(* Logix 5000 Rung export; software revision 16.04 *)

MODULES
   Local : vendor None type None code None
   MVI69E_AFC : vendor None type None code None
END_MODULES

TYPE AFCESiteAlarms :   // Indicates if a meter has any alarms
STRUCT
   Meter1 : BOOL;   // Meter in alarm
   Meter2 : BOOL;   // Meter in alarm
   Meter3 : BOOL;   // Meter in alarm
   Meter4 : BOOL;   // Meter in alarm
   Meter5 : BOOL;   // Meter in alarm
   Meter6 : BOOL;   // Meter in alarm
   Meter7 : BOOL;   // Meter in alarm
   Meter8 : BOOL;   // Meter in alarm
   Meter9 : BOOL;   // Meter in alarm
   Meter10 : BOOL;   // Meter in alarm
   Meter11 : BOOL;   // Meter in alarm
   Meter12 : BOOL;   // Meter in alarm
   Meter13 : BOOL;   // Meter in alarm
   Meter14 : BOOL;   // Meter in alarm
   Meter15 : BOOL;   // Meter in alarm
   Meter16 : BOOL;   // Meter in alarm
END_STRUCT
END_TYPE

TYPE AFCEMeterDifferentialGasBackPlaneReturn :   // Differential Gas Meter
STRUCT
   StandardDefault : AFCEMeterDifferentialGasStandardDataDflt;
   StandardRaw : INT[14];
   Extended : AFCEExtended;
END_STRUCT
END_TYPE

TYPE AFCEFlag :   // Flags contains status information updated by ladder and also trigger bits for clock update
STRUCT
   AFCStopped : BOOL;   // Indicates that the module has sent a new input block to be processed by ladder - UPDATED BY LADDER
   AFCInputSequenceNum : INT;   // Meter number (0 -15) associated to blocks 1-16. Used to update "Profile" (meter type and product group.) UPDATED BY LADDER
END_STRUCT
END_TYPE

TYPE AFCEUtilBlockNonInterrupt :
STRUCT
   Now : BOOL;
   ModbusMasterCommand : BOOL;
   ModbusMasterResponse : BOOL;
   Archive : DINT;
   Prover : BOOL;
   PassThru : BOOL;
   Calibration : BOOL;
END_STRUCT
END_TYPE

TYPE AFCEMeterDifferentialGasArchiveWrite :   // Write Archive
STRUCT
   Daily : BOOL;   // Set to 1 to write daily archive
   Hourly : BOOL;   // Set to 1 to write hourly archive
END_STRUCT
END_TYPE

TYPE AFCEMeterCalRequestActionType :
STRUCT
   ZeroShift : BOOL;   // Zero Shift
   SetZero : BOOL;   // Set Zero
   SetSpan : BOOL;   // Set Span
   SetMid1 : BOOL;   // Set Mid 1
   SetMid2 : BOOL;   // Set Mid 2
   SetMid3 : BOOL;   // Set Mid 3
END_STRUCT
END_TYPE

TYPE AFCEProveConfigEnable :   // Prove controls at enable
STRUCT
   MeterNumber : INT;   // Meter number requested (1-16)
   AutoAcceptProve : BOOL;   // Auto-accept the prove
   AutoContinueProve : BOOL;   // Auto-continue the prove
END_STRUCT
END_TYPE

TYPE AFCEModbusGateway :   // Modbus Gateway
STRUCT
   Command : AFCEModbusGatewayCommand[10];   // Modbus gateway commands - contains setup and modbus data
END_STRUCT
END_TYPE

TYPE AFCEMeterCalRequestActionValue :
STRUCT
   ZeroShift : AFCEMeterCalRequestValue;   // Zero Shift
   SetZero : AFCEMeterCalRequestValue;   // Set Zero
   SetSpan : AFCEMeterCalRequestValue;   // Set Span
   SetMid1 : AFCEMeterCalRequestValue;   // Set Mid 1
   SetMid2 : AFCEMeterCalRequestValue;   // Set Mid 2
   SetMid3 : AFCEMeterCalRequestValue;   // Set Mid 3
END_STRUCT
END_TYPE

TYPE AFCEMeterAnalysisError :
STRUCT
   StreamOutOfRange : BOOL;   // Requested Stream Number Out of Range
   StreamNotConfigured : BOOL;   // Requested Stream Not Configured
END_STRUCT
END_TYPE

TYPE AFCEMeterCalRequestValue :
STRUCT
   Applied : REAL;   // Applied
   Measured : REAL;   // Measured
END_STRUCT
END_TYPE

TYPE AFCEModbusMasterDataType :   // Modbus master data type
STRUCT
   Bit : BOOL;   // bit type
   Word : BOOL;   // word type (16-bit)
   Long : BOOL;   // long integer (32-bit)
   LongRemote : BOOL;   // long integer (32-bit)
END_STRUCT
END_TYPE

TYPE AFCEUtil :   // Used for internal ladder logic usage. These values must not be changed by user application.
STRUCT
   Flags : AFCEFlag;   // Wallclock update commands
   CycleCounter : INT;   // Reflects current block ID calculated by ladder to be sent to the module
   Buffer : AFCEUtilBuffer;
   Block : AFCEUtilBlock;
END_STRUCT
END_TYPE

TYPE AFCEWallclock :
STRUCT
   GetAFCTime : BOOL;   // Get current AFC Time
   SetAFCTimeFromPLCTime : BOOL;   // Set AFC time from PLC time. Updates current AFC time
   EnableLocalDateTime : BOOL;   // Enable Local Date Time.
   AFCTime : AFCETime;   // Coordinated Universal Time. Updated by either getting or setting AFC time.
END_STRUCT
END_TYPE

TYPE AFCEProvePhaseBitmap :   // AFC prove phase bitmap
STRUCT
   NotSelected : BOOL;   // Not selected
   Active : BOOL;   // Active, not counting
   CountingPast1stSwitch : BOOL;   // Counting past 1st switch for Udir and forward leg for Bdir)
   Past2ndSwitchFwdLeg : BOOL;   // Past 2nd switch forward leg (bidirectional only)
   Past1stSwithRetLeg : BOOL;   // Past 1st switch return leg (bidirectional only)
   RunComplete : BOOL;   // Run complete. past 2nd switch.
END_STRUCT
END_TYPE

TYPE AFCEProveInputConfig :   // Prove input block results - prover configuration
STRUCT
   Type : INT;   // Prover type
   Options : INT;   // Prover options
   RunsPerProveTotal : INT;   // Total runs per prove
   RunsPerProveSelected : INT;   // Selected runs per prove
   MaxRunsBeforeAbort : INT;   // Max total runs before abort
   ShortPassesPerRun : INT;   // Short passes per run if bidir = 2 , else 0
END_STRUCT
END_TYPE

TYPE AFCEMeterCalResponse :
STRUCT
   Trigger : BOOL;   // Send Error Code and Values to module to be recorded
   ErrorCode : SINT;   // Error Code to send. 0-4 allowed. 0=No error. 1-4=User defined.
   Value : AFCEMeterCalRequestValue;   // Value to Send
   Count : DINT;   // Number of calibration responses
END_STRUCT
END_TYPE

TYPE AFCEMeterDifferentialGasArchive :   // Different Gas Archive
STRUCT
   Write : AFCEMeterDifferentialGasArchiveWrite;
   Fetch : AFCEMeterDifferentialGasArchiveFetch;
END_STRUCT
END_TYPE

TYPE AFCEMeterDifferentialGasArchiveDflt :   // Default Configuration
STRUCT
   ClosingTimestamp : DINT;
   CumulativeActiveStreams : INT;
   CurrentActiveStream : SINT;
   MeterStatus : SINT;
   FlowingPeriod : DINT;
   PeriodDuration : DINT;
   AccumulatorTotalizer : DINT;
   AccumulatorResidue : REAL;
   MeterAlarms : DINT;
   PrimaryInput : REAL;   // Either Differential Pressure or Flow Rate
   Temperature : REAL;
   Pressure : REAL;
   RelativeDensity : REAL;
   ReferenceCompressibility : REAL;
   FlowingCompressibility : REAL;
   Fpv : REAL;
   PressureExtension : REAL;
   CoefficientDischarge : REAL;
   ExpansionFactor : REAL;
   Cprime : REAL;
   MassNRAccumulatorCurrent : REAL;   // Non-resettable
   MassNRAccumulatorOpening : REAL;   // Non-resettable
   EnergyNRAccumulatorCurrent : REAL;   // Non-resettable
   EnergyNRAccumulatorOpening : REAL;   // Non-resettable
   NetNRAccumulatorCurrent : REAL;   // Non-resettable
   NetNRAccumulatorOpening : REAL;   // Non-resettable
   GrossNRAccumulatorCurrent : REAL;   // Non-resettable
   GrossNRAccumulatorOpening : REAL;   // Non-resettable
   MolarFractionComponent01_C1 : REAL;
   MolarFractionComponent02_N2 : REAL;
   MolarFractionComponent03_CO2 : REAL;
   MolarFractionComponent04_C2 : REAL;
   MolarFractionComponent05_C3 : REAL;
   MolarFractionComponent06_H2O : REAL;
   MolarFractionComponent07_H2S : REAL;
   MolarFractionComponent08_H2 : REAL;
   MolarFractionComponent09_CO : REAL;
   MolarFractionComponent10_O2 : REAL;
   MolarFractionComponent11_IC4 : REAL;
   MolarFractionComponent12_NC4 : REAL;
   MolarFractionComponent13_IC5 : REAL;
   MolarFractionComponent14_NC5 : REAL;
   MolarFractionComponent15_C6 : REAL;
   MolarFractionComponent16_C7 : REAL;
   MolarFractionComponent17_C8 : REAL;
   MolarFractionComponent18_C9 : REAL;
   MolarFractionComponent19_C10 : REAL;
   MolarFractionComponent20_He : REAL;
   MolarFractionComponent21_Ar : REAL;
   UserDefinedFlowAverage1 : REAL;
   UserDefinedFlowAverage2 : REAL;
   UserDefinedFlowAverage3 : REAL;
END_STRUCT
END_TYPE

TYPE AFCEMeterDifferentialGasAlarm :   // Alarm Status and Control
STRUCT
   Control : AFCEMeterDifferentialGasAlarmControl;   // Alarm Control
END_STRUCT
END_TYPE

TYPE AFCEMeterDifferentialGasArchiveFetch :
STRUCT
   Daily : AFCEMeterDifferentialGasArchiveFetchT;
   Hourly : AFCEMeterDifferentialGasArchiveFetchT;
END_STRUCT
END_TYPE

TYPE AFCEMeterDifferentialGasAlarmControl :   // Differential Gas Process Alarm Control
STRUCT
   DifferentialPressure : AFCEMeterProcessAlarm;   // Differential Pressure Alarms
   FlowRate : AFCEMeterProcessAlarm;   // Flow Rate
   Temperature : AFCEMeterProcessAlarm;   // Temperature Alarms
   Pressure : AFCEMeterProcessAlarm;   // Pressure Alarms
END_STRUCT
END_TYPE

TYPE AFCEMeterArchiveFetchError :
STRUCT
   ArchiveSelectionInvalid : BOOL;   // Archive File Selection Invalid
   AgeOutsideSize : BOOL;   // Age Outside Configured File Size
   ArchiveNeverWritten : BOOL;   // Age OK but Archive Record Never Written (new or reconfigured meter)
   Reserverd1 : BOOL;
   Reserverd2 : BOOL;
   Reserverd3 : BOOL;
   Reserverd4 : BOOL;
   Reserverd5 : BOOL;
   Reserverd6 : BOOL;
   Reserverd7 : BOOL;
   Reserverd8 : BOOL;
   Reserverd9 : BOOL;
   Reserverd10 : BOOL;
   Reserverd11 : BOOL;
   Reserverd12 : BOOL;
   Reserverd13 : BOOL;
END_STRUCT
END_TYPE

TYPE AFCEModbusGatewayCommand :   // Modbus Gateway Command
STRUCT
   Config : AFCEModbusGatewayConfig;   // Config data to be entered by the user.
   Trigger : BOOL;   // Trigger the Command, when cleared module has responded.
   Data : INT[200];   // Contains modbus data written to the module (write commands)
END_STRUCT
END_TYPE

TYPE AFCEProveConfigAccept :   // Prove controls at accept. If auto-accept is selected must be available at enable
STRUCT
   RequestedInterpolationPoint : INT;   // Requested interpolation point (0 nearest)
   ApplyMFChangeAllStreams : BOOL;   // Apply change in meter factor to all streams
   ApplyMFChangeCurve : BOOL;   // Apply change in meter factor to all curve points
   ApplyNewMF : BOOL;   // CApply new meter factor
END_STRUCT
END_TYPE

TYPE AFCEModbusMasterCommand :   // Modbus Master Command
STRUCT
   Config : AFCEModbusMasterConfig;   // Modbus Master Configuration
   ErrorCode : INT;   // Error Code associated to Modbus Master Command
   Pending : BOOL;   // Pending Modbus Master Command - waiting for Modbus Response
   ReturnedTransactionID : DINT;   // Changes to Config.TransactionID value when response has returned.
   Data : INT[100];   // Read or Write Data
END_STRUCT
END_TYPE

TYPE AFCEMeterStatusMeter :   // Meter Status
STRUCT
   Enabled : BOOL;   // Meter Enable Status, 1=enabled
   EnableAlarm : BOOL;   // If set either: 1. The meter is not configured. 2. The event log is full, the action was not performed.
END_STRUCT
END_TYPE

TYPE AFCEMeterControl :   // Enable/Disable Meter and Streams
STRUCT
   Meter : AFCEMeterControlMeter;   // Control the Meter
   Stream : AFCEMeterControlStream;   // Control the Meter Streams
   ResetAccumulators : AFCEMeterSignals;   // Resets for meter accumulators
END_STRUCT
END_TYPE

TYPE AFCEProveSequencing :   // AFC prove sequencing tag for phase selection and ball positioning
STRUCT
   Phase : AFCEProvePhaseBitmap;   // AFC phase sequencing
   BallPositionReady : BOOL;   // Ball position: Ready (Udir & Bdir only; fwd leg Bdir)
   BallPositionSealed : BOOL;   // Ball position: Sealed (Udir & Bdir only; fwd leg Bdir)
   BallPositionReadyBwdLeg : BOOL;   // Ball position: Ready bwd leg (Bdir only)
   BallPositionSealedBwdLeg : BOOL;   // Ball position: Sealed bwd leg (Bdir only)
END_STRUCT
END_TYPE

TYPE AFCEMeterDifferentialGasArchiveFetchT :   // Fetch Archive
STRUCT
   Trigger : BOOL;   // Trigger Archive Fetch
   Age : INT;   // Initial Archive. 0 = Current Archive
   Error : AFCEMeterArchiveFetchError;   // Archive Fetch Error
   Default : AFCEMeterDifferentialGasArchiveDflt;   // Default Archive
   Raw : INT[100];   // Raw Archive
END_STRUCT
END_TYPE

TYPE AFCEUtilBlockInterrupt :
STRUCT
   Now : BOOL;
   ModbusGateway : DINT;
   EnableDisable : BOOL;
   Analysis : DINT;
END_STRUCT
END_TYPE

TYPE AFCEComponents :   // High precision gas component analysis (only supported version 2.07.000)
STRUCT
   C1 : REAL;   // Methane
   N2 : REAL;   // Nitrogen
   CO2 : REAL;   // Carbon Dioxide
   C2 : REAL;   // Ethane
   C3 : REAL;   // Propane
   H20 : REAL;   // Water
   H2S : REAL;   // Hydrogen Sulphide
   H2 : REAL;   // Hydrogen
   CO : REAL;   // Carbon Monoxide
   O2 : REAL;   // Oxygen
   IC4 : REAL;   // Iso-butane
   NC4 : REAL;   // Normal Butane
   IC5 : REAL;   // Iso-pentane
   NC5 : REAL;   // Normal-pentane
   C6 : REAL;   // Hexane
   C7 : REAL;   // Heptane
   C8 : REAL;   // Octane
   C9 : REAL;   // Nonane
   C10 : REAL;   // Decane
   He : REAL;   // Helium
   Ar : REAL;   // Argon
   NeoC5 : REAL;   // Not Used
   UxUser1 : REAL;   // Not Used
   UyUser2 : REAL;   // Not Used
   UxUser3 : REAL;   // Not Used
   UyUser4 : REAL;   // Not Used
   UxUser5 : REAL;   // Not Used
   UyUser6 : REAL;   // Not Used
   UxUser7 : REAL;   // Not Used
   UyUser8 : REAL;   // Not Used
   UxUser9 : REAL;   // Not Used
   UyUser10 : REAL;   // Not Used
END_STRUCT
END_TYPE

TYPE AFCEMeterStatus :   // Status
STRUCT
   Meter : AFCEMeterStatusMeter;   // Meter Status
   Stream : AFCEMeterStatusStream;   // Stream Status
END_STRUCT
END_TYPE

TYPE AFCEUtilBlock :
STRUCT
   ProcessInput : INT;
   InterruptPending : AFCEUtilBlockInterrupt;
   InterruptComplete : AFCEUtilBlockInterrupt;
   NonInterruptPending : AFCEUtilBlockNonInterrupt;
   NonInterruptComplete : AFCEUtilBlockNonInterrupt;
END_STRUCT
END_TYPE

TYPE AFCEModbusGatewayConfig :   // Modbus Ggateway Configuration
STRUCT
   Enable : BOOL;   // Set to 1 to enable modbus gateway command (0=disable)
   StartRegister : DINT;   // Start modbus address
   RegisterCount : INT;   // Word count (200 max)
   FunctionType : BOOL;   // 0 = read command, 1 = write command
   RegisterType : BOOL;   // 0 = holding register, 1 = input register
   SlaveType : BOOL;   // 0 = primary slave, 1 = virtual slave
END_STRUCT
END_TYPE

TYPE AFCEMeterControlMeter :   // Enable and Disable Meter
STRUCT
   Enable : BOOL;   // Enable the Meter
   Disable : BOOL;   // Disable the Meter
END_STRUCT
END_TYPE

TYPE AFCEMeterProfile :   // Meter configuration profile
STRUCT
   MeterType : BOOL;   // 0=Differential, 1=Linear
   ProductGroup : BOOL;   // 0=Gas, 1=Liquid
   PrimaryInput : BOOL;   // For differential, 0=Differential Pressure 1=Flow Rate. For Linear, 0=Pulse Count 1=Pulse Frequency
   AOIMismatch : BOOL;   // AOI Meter type does not match module for meter number
END_STRUCT
END_TYPE

TYPE AFCEModbusPassThru :   // AFC Modbus Pass-thru
STRUCT
   Enable : BOOL;   // Set to 1 to enable pass-thru functionality (requires AFC Manager setting)
   MessagePresent : BOOL;   // Message present in the response block
   GetMessage : BOOL;   // Get the pass-thru message. When the bit is cleared the message has been transferred to the PLC.
   FunctionBitWrite : BOOL;   // Function bit write
   OverflowError : BOOL;   // Overflow error flag
   ModbusAddress : INT;   // Destination modbus address
   RegisterCount : INT;   // Number of elements associated to command
   ReadDataWord : INT[125];   // Contains received data for word commands
   ReadDataBit : AFCEModbusPassThruBitData;   // Contains received data for bit commands
END_STRUCT
END_TYPE

TYPE AFCEUtilBuffer :   // Buffer
STRUCT
   Input : INT[248];   // Input buffer contains the complete block to be copied from the module
   Output : INT[247];   // Output buffer contains data the complete block to be copied to the module
   Process : INT[180];
   ArchiveDay : INT[98];
   ArchiveHour : INT[98];
   Prove : INT[26];
   Analysis : INT[198];
   MeterEnableDisable : INT[4];
   StreamEnable : INT[36];
   StreamDisable : INT[36];
   StreamSelect : INT[24];
   MeterSignals : INT[24];
   Calibration : INT[36];
END_STRUCT
END_TYPE

TYPE AFCEMeterDifferentialGasCalRequestProces :
STRUCT
   DifferentialPressure : BOOL;   // Differential Pressure
   Temperature : BOOL;   // Temperature
   Pressure : BOOL;   // Pressure
END_STRUCT
END_TYPE

TYPE AFCEProveStatus :   // Status of the prove (returned from the module to the processor)
STRUCT
   ProveAccepted : BOOL;   // Prove was accepted
   MeterFactorApplied : BOOL;   // Meter factor was applied
   MFAppliedToCurve : BOOL;   // Meter factor was applied to all points in the curve
   MFAppliedToStreams : BOOL;   // Meter factor was applied to all streams
   ProveRejectedByCommand : BOOL;   // Prove was rejected by command
   ProveRejectedNoRuns : BOOL;   // Prove was rejected - empty prove (no runs)
   ProveRejectedDivideBy0 : BOOL;   // Prove was rejected - divide by 0
   ProveEnabled : BOOL;   // Prove is enabled
   ProvingRunInProgress : BOOL;   // Proving run is in progress
   ProveRejectedAbort : BOOL;   // Prove rejected: abort
   ProvePaused : BOOL;   // Prove is paused
   RunCancelled : BOOL;   // Run Is cancelled
   RunTimedOut : BOOL;   // Run timed out
END_STRUCT
END_TYPE

TYPE AFCEMeterStatusStreamAlarm :   // Stream Alarms
STRUCT
   StreamOutOfRange : BOOL;   // Requested Stream Number Out of Range
   StreamNotConfigured : BOOL;   // Requested Stream not Configured
   StreamNotEnabled : BOOL;   // Requested Stream not Enabled
   EventLogFull : BOOL;   // Event Log Full, Action not Performed
END_STRUCT
END_TYPE

TYPE AFCEMeterDifferentialGasCalRequest :
STRUCT
   ProcessVariable : AFCEMeterDifferentialGasCalRequestProces;   // Process Variable
   ActionType : AFCEMeterCalRequestActionType;   // Action Type
   Value : AFCEMeterCalRequestActionValue;   // Value
   Count : DINT;   // Number of calibration requests
END_STRUCT
END_TYPE

TYPE AFCEProveConfig :   // Controls (configuration settings) associated to the prover
STRUCT
   Enable : AFCEProveConfigEnable;   // Controls at enable
   Accept : AFCEProveConfigAccept;   // Controls at accept
END_STRUCT
END_TYPE

TYPE AFCESiteStatus :   // Site status bits - contains general information about the module - not meter specific
STRUCT
   AFCActive : BOOL;   // AFC active
   ChecksumAlarms : BOOL;   // Checkum alarm active
   Reserved2 : BOOL;
   Reserved3 : BOOL;
   PLCHalted : BOOL;   // PLC in program mode or missing
   CfgChanged : BOOL;   // Configuration changed
   Powerup : BOOL;   // Module powered up
   ColdStart : BOOL;   // Module performed cold start (BBRAM initialized)
   ModbusMasterPending : BOOL;   // Modbus Master Poll Pending
   ModbusMasterComplete : BOOL;   // Modbus Master Poll Complete
   ModbusPassThruPending : BOOL;   // Modbus Pass-thru Input Pending
   CalibrationRequest : BOOL;   // Calibration request from module
   ProverEnabled : BOOL;   // Prover Enabled
   Reserved13 : BOOL;
   Reserved14 : BOOL;
   Reserved15 : BOOL;
END_STRUCT
END_TYPE

TYPE AFCEMeterDifferentialGasStandardDataDflt :   // EAFC Backplane Return Standard Data
STRUCT
   Meter_Alarms : DINT;   // Meter alarms
   NR_Acc_Net_Totalizer : DINT;   // Non-resettable accumulator, net, totalizer (m3)
   NR_Acc_Net_Residue : REAL;   // Non-resettable accumulator, net, residue (m3)
   FlowRate_Net : REAL;   // Flow rate, net (m3/h)
   FlowRate_Gross : REAL;   // Flow rate, gross (m3/h)
   Ifpv : REAL;   // AGA 8, Supercompressibility, Fpv
   Cprime : REAL;   // C-prime
END_STRUCT
END_TYPE

TYPE AFCEModbusMaster :   // Modbus Master. Port 3 must be configured as modbus master through AFC Manager to use this feature.
STRUCT
   Enable : BOOL;   // Enable the modbus master funcionality
   CommandIndex : INT;   // Selects which command index will be executed
   Command : AFCEModbusMasterCommand[10];   // Each command contains a specific modbus request to be sent out of the port
END_STRUCT
END_TYPE

TYPE AFCEProveProcess :   // Prove process output from processor to the module
STRUCT
   Sequencing : AFCEProveSequencing;   // Prover sequencing
   Temperature : REAL;   // Temperature for Single Probe provers. And Inlet Temperature for Dual Probe Provers.
   OutletTemperature : REAL;   // Outlet Temperature for Provers with Dual Probes.
   SwitchBarTemperature : REAL;   // Switch bar temperature
   Pressure : REAL;   // Pressure for Single Probe provers. And Inlet Pressure for Dual Probe Provers.
   OutletPressure : REAL;   // Outlet Pressure for Provers with Dual Probes.
   ProverDensity : REAL;   // Prover density
END_STRUCT
END_TYPE

TYPE AFCEExtended :
STRUCT
   Trigger : BOOL;
   Data : AFCEExtendedData;
END_STRUCT
END_TYPE

TYPE AFCEMeterSignals :   // Meter trigger accumulator and archive resets
STRUCT
   ResetAccumulator1 : BOOL;   // Set to 1 to reset resettable accumulator 1
   ResetAccumulator2 : BOOL;   // Set to 1 to reset resettable accumulator 2
   ResetAccumulator3 : BOOL;   // Set to 1 to reset resettable accumulator 3
   ResetAccumulator4 : BOOL;   // Set to 1 to reset resettable accumulator 4
END_STRUCT
END_TYPE

TYPE AFCEMeterProcessAlarm :   // Process Alarms
STRUCT
   SetGeneralFail : BOOL;   // Set to indicate General Failure of the Transmitter
   StaleData : BOOL;   // Clear to Indicate new process input data
   SetLowThreshold : BOOL;   // Set to indicate Lower Range Limit Exceeded
   SetHighThreshold : BOOL;   // Set to indicate Upper Range Limit Exceeded
   SetAutoClearStaleData : BOOL;   // Set to automatically clear stale data
END_STRUCT
END_TYPE

TYPE AFCETime :   // AFC time format used for wallclock update.
STRUCT
   Year : DINT;   // Year
   Month : DINT;   // Month
   Day : DINT;   // Day
   Hour : DINT;   // Hour
   Minute : DINT;   // Minute
   second : DINT;   // Seconds
END_STRUCT
END_TYPE

TYPE AFCEModbusMasterSwap :   // Modbus master swap words/ swap bytes
STRUCT
   SwapWords : BOOL;   // Swap words
   SwapBytes : BOOL;   // Swap bytes
END_STRUCT
END_TYPE

TYPE AFCEMeterControlStream :
STRUCT
   Selected : SINT;   // Stream to Enable or Disable and/or make active.
   EnableSelected : BOOL;   // Enable the Selected Stream
   DisableSelected : BOOL;   // Disable the Selected Stream
   SetSelectedToActive : BOOL;   // Set Selected to Active Stream
END_STRUCT
END_TYPE

TYPE AFCEProvePulseCount :   // Values to be supplied at the end of the pass/run
STRUCT
   Meter : DINT;   // Meter pulse count
   MasterMeter : DINT;   // Master meter pulse count
END_STRUCT
END_TYPE

TYPE AFCEMeterDifferentialGasCal :   // Processor Mediated Calibration
STRUCT
   Request : AFCEMeterDifferentialGasCalRequest;   // Calibration Request from module
   Response : AFCEMeterCalResponse;   // Processor Response
END_STRUCT
END_TYPE

TYPE AFCEMeterStatusStream :
STRUCT
   Active : INT;   // Current Active Stream
   Enabled : AFCEMeterStatusStreamEnabled;   // Enabled Streams
   Configured : AFCEMeterStatusStreamEnabled;   // Configured Streams
   EnableAlarm : AFCEMeterStatusStreamAlarm;   // Enable Alarms
END_STRUCT
END_TYPE

TYPE AFCEExtendedData :
STRUCT
   Raw : INT[64];
END_STRUCT
END_TYPE

TYPE AFCEMeterDifferentialGasProcess :   // Differential Gas Process Variables
STRUCT
   DifferentialPressure : REAL;   // Differential pressure if Primary Input = Differential pressure
   FlowRate : REAL;   // Flow Rate if Primary Input = Flow Rate
   Temperature : REAL;   // Temperature
   Pressure : REAL;   // Static pressure
END_STRUCT
END_TYPE

TYPE AFCEModbusPassThruBitData :   // AFC Modbus Pass-thru Bit Data
STRUCT
   Data : BOOL[2016];   // Contains received data for bit commands
END_STRUCT
END_TYPE

TYPE AFCEModbusMasterConfig :   // Modbus master command settings
STRUCT
   Enable : BOOL;   // Set to 1 to enable command (0=disable)
   FunctionType : BOOL;   // Set to 1 to select write command (0=read command)
   RegisterBank : BOOL;   // Set to 1 to select input register (0=holding register)
   DataType : AFCEModbusMasterDataType;   // Select data type format
   SwapOption : AFCEModbusMasterSwap;   // Select byte and word swap (1 = swap, 0 = no swap)
   TypeSwap : INT;   // This value is calculated by ladder logic and must not be modified by user
   SlaveAddress : INT;   // Modbus slave address of remote device
   ModbusAddress : INT;   // Modbus data address on remote slave
   ElementCount : INT;   // Number of data elements (125 words)
   TransactionID : INT;   // Transaction ID. This value is returned to the ReturnedTransaction ID when the response has been received.
END_STRUCT
END_TYPE

TYPE AFCEModuleDef :   // Main user defined data type
STRUCT
   ModbusGateway : AFCEModbusGateway;   // Reads and write data between processor and module modbus table
   ModbusMaster : AFCEModbusMaster;   // Setup modbus master commands to be sent to remote slaves (through Port 3)
   ModbusPassThru : AFCEModbusPassThru;   // Modbus pass-thru data
   SiteStatus : AFCESiteStatus;   // Site status
   MeterAlarms : AFCESiteAlarms;   // Meter Alarms
   Prove : AFCEProve;   // Prover
   Wallclock : AFCEWallclock;   // Set clock and get clock information
   Firmware : AFCEFirmwareVersion;   // Firmware information
   Util : AFCEUtil;   // Used by ladder logic
END_STRUCT
END_TYPE

TYPE AFCEMeterDifferentialGas :   // Differential Gas Meter
STRUCT
   Control : AFCEMeterControl;   // Meter Control
   Status : AFCEMeterStatus;   // Meter Status
   ProcessVariables : AFCEMeterDifferentialGasProcess;   // Input process variables to be transferred to the module
   Analysis : AFCEMeterAnalysis;   // Molar Analysis data to be transferred to the module (only for gas products with online gas chromatograph applications)
   Alarm : AFCEMeterDifferentialGasAlarm;   // Meter Alarm status and control
   Archive : AFCEMeterDifferentialGasArchive;   // Archive
   Profile : AFCEMeterProfile;   // Module profile (meter type/product group) transfered from the module
   Calibration : AFCEMeterDifferentialGasCal;   // Calibration
   BackPlaneReturn : AFCEMeterDifferentialGasBackPlaneReturn;
END_STRUCT
END_TYPE

TYPE AFCEMeterAnalysis :   // Meter analysis components. Allows the processor to update molar analysis for low precision and high precision streams.
STRUCT
   Trigger : BOOL;   // Set to 1 to Send Updated Component Data to the Module
   Stream : INT;   // Stream for Analysis. Select 0 for current active stream.
   Error : AFCEMeterAnalysisError;   // Analysis Error
   Components : AFCEComponents;   // High precision gas components (floating point per component). Only supported for firmware version 2.07.000 or later
END_STRUCT
END_TYPE

TYPE AFCEProveSignals :   // Contains the proving signals that will trigger specific tasks from the module
STRUCT
   EnableProve : BOOL;   // Enables the prove
   AcceptProve : BOOL;   // Accepts the prove
   RejectProve : BOOL;   // Reject the prove
   RunStart : BOOL;   // Starts the run
   RunComplete : BOOL;   // Flags that the run is complete
   RunCancel : BOOL;   // Cancels the run
   RunDelete : BOOL;   // Deletes the run
   PassComplete : BOOL;   // Flag that the pass is complete
   PauseProve : BOOL;   // Pauses the Proving Process
   AbortProve : BOOL;   // Aborts the prove
END_STRUCT
END_TYPE

TYPE AFCEFirmwareVersion :
STRUCT
   Major : SINT;   // Major Version number
   Minor : SINT;   // Minor Version number
   Revision : INT;   // Revision
END_STRUCT
END_TYPE

TYPE AFCEProveRunResults :   // Run results of the prove. Copied from the module to the pocessor
STRUCT
   CountAttempted : INT;   // Run count attempted
   CountCompleted : INT;   // Run count completed
   CountSelected : INT;   // Run count selected
   RunsSelected : INT;   // Bit Mapped Runs selected for calculations from completed runs
   NewMeterFactor : REAL;   // New meter factor
   ChangeInMeterFactor : REAL;   // Change in meter factor
END_STRUCT
END_TYPE

TYPE AFCEMeterStatusStreamEnabled :   // Stream Status 1 = Enabled
STRUCT
   Stream1 : BOOL;
   Stream2 : BOOL;
   Stream3 : BOOL;
   Stream4 : BOOL;
   Stream5 : BOOL;
   Stream6 : BOOL;
   Stream7 : BOOL;
   Stream8 : BOOL;
   Stream9 : BOOL;
   Stream10 : BOOL;
   Stream11 : BOOL;
   Stream12 : BOOL;
   Stream13 : BOOL;
   Stream14 : BOOL;
   Stream15 : BOOL;
   Stream16 : BOOL;
END_STRUCT
END_TYPE

TYPE AFCEProve :   // Prove
STRUCT
   Process : AFCEProveProcess;   // Process Variables
   Signals : AFCEProveSignals;   // AFC Prove Signals (triggers the proving update)
   Config : AFCEProveConfig;   // AFC Prove Control (configuration settings)
   PulseCounts : AFCEProvePulseCount;   // Pulse counts to be updated at the end of the run/pass
   ConfigInput : AFCEProveInputConfig;   // AFC prover input configuration
   Status : AFCEProveStatus;   // AFC prover status
   ErrorCode : INT;   // Prove error code
   ProveControlsEcho : INT;   // AFC module Echos the state of the Prove Controls
   RequestedMeterEcho : INT;   // AFC module Echos the Meter number requested
   RequestedCurvePointEcho : INT;   // AFC module Echos the requested Curve Point
   RunResults : AFCEProveRunResults;   // Prove and run results
   ProveEnabled : BOOL;   // ON if prove is enabled. This flag is coped from inputbuffer[247]
END_STRUCT
END_TYPE

ADD_ON_INSTRUCTION AOI69EAFCMeterDifferentialGas   (* revision 1.6, vendor ProSoft Technology Inc., ExecutePrescan *)
// Add-On instruction for the MVI69E-AFC.
// Differential Gas Meter
// Revision note:
// Updated  BackplaneReturn Tag name from ProcessInputs to Standard
// and ComponentAnalysis to Extended
// Help:
// AOI69EAFCMeterDifferentialGas v1.1
// Compatible with version 4.04 of MVI69E-AFC firmware or higher.
// v1.1 Comp Analysis Return fix
// v1.2 Added Flow Rate Process Input and Flow Rate Alarm Controller Tags for Flow Rate Devices (and not just for Differential Pressure)
// v1.3: Addition of default process input backplane return data mapping..
// v1.4: Changed Prescan FLL instruction length from 240 words to 180 for proccess inputs. This stopped mismatch issue
// v1.4:  Made correlation changes between the Module Archive Default UDTs and the AOI Archive Default UDTs.
// v1.5: Made changes to the Flow Rate Primary Input Block ID Insertion in Rung 8 (Removed +1), Modified ProcessInputBlockID Tag Data Type from DINT to INT and modified ModbusGatewayConfig UDT StartRegister Tag Data Type from INT to DINT.
// v1.6: Updated Tags names AFCMeterXXYYYYYY.BackPlaneReturn.ProcessInputs to
// AFCMeterXXYYYYYY.BackPlaneReturn.Standard and
// AFCMeterXXYYYYYY.BackPlaneReturn.ComponentAnalysis
//  to AFCMeterXXYYYYYY.BackPlaneReturn.Extended.
VAR_IN_OUT
   ConnectionInput : INT[248]; {required}
   AFC : AFCEModuleDef; {required}
   AFCMeter : AFCEMeterDifferentialGas; {required}
END_VAR
VAR_INPUT
   MeterNumber : SINT; {required}   // Meter Number Set to a number between 1 and 16
END_VAR
VAR
   TimestampBuffer : DINT;
   StreamSelectedShift : DINT;
   StreamSelectBuffer : INT;
   EnabledStatusBuffer : INT;
   StreamSelectBlockID : DINT;
   StreamNumberShift : DINT;
   StreamErrorBuffer : DINT;
   StreamEnableBlockID : DINT;
   StreamEnableBitPosition : DINT;
   StreamDisableBlockID : DINT;
   ProfileBuffer : SINT[2];
   ProcessInputBlockID : DINT;
   CalibrationHandleBuffer : INT;
   AnalysisGroupBitPosition : INT;
   ProcessAlarmShifter : DINT;
   ProcessAlarmBuffer : DINT;
   MeterSignaltBlockID : DINT;
   MeterNumberShift : DINT;
   MeterNumberBitPostition : DINT;
   Inputbuffer : INT[248];
   CurrentHourlyAgeONS : BOOL;
   CurrentHourlyAge : DINT;
   CurrentDailyAgeONS : BOOL;
   CurrentDailyAge : DINT;
   ClearMeterSignal : BOOL;   // Repeat the meter signal block with cleared signal bits. This allows repeat triggering of a signal.
   CalibrationMeterNumberBuffer : DINT;
   CalibrationMediationPending : BOOL;
   CalibrationInputScalingIndex : DINT;
   AnalysisErrorBuffer : INT;
   ArchiveStream : DINT;
   ArchiveMeterStatusRaw : DINT;
   ArchiveMeterStatusActiveStream : DINT;
   ArchiveHourlyRawSize : DINT;
   ArchiveHourlyOffset : DINT;
   ArchiveHourlyDefaultSize : DINT;
   ArchiveDailyRawSize : DINT;
   ArchiveDailyOffset : DINT;
   ArchiveDailyDefaultSize : DINT;
   ArchiveCompleteBitCheck : DINT;
   ArchiveBlockID : DINT;
   AnalysisGroupShift : DINT;
   AnalysisCompleteBitCheck : DINT;
   AnalysisBufferOffset : DINT;
   AnalysisBlockID : DINT;
   AFCStopped : BOOL;
   AFCInputDataAvailable : BOOL;
END_VAR

ROUTINE Logic   (* ladder *)
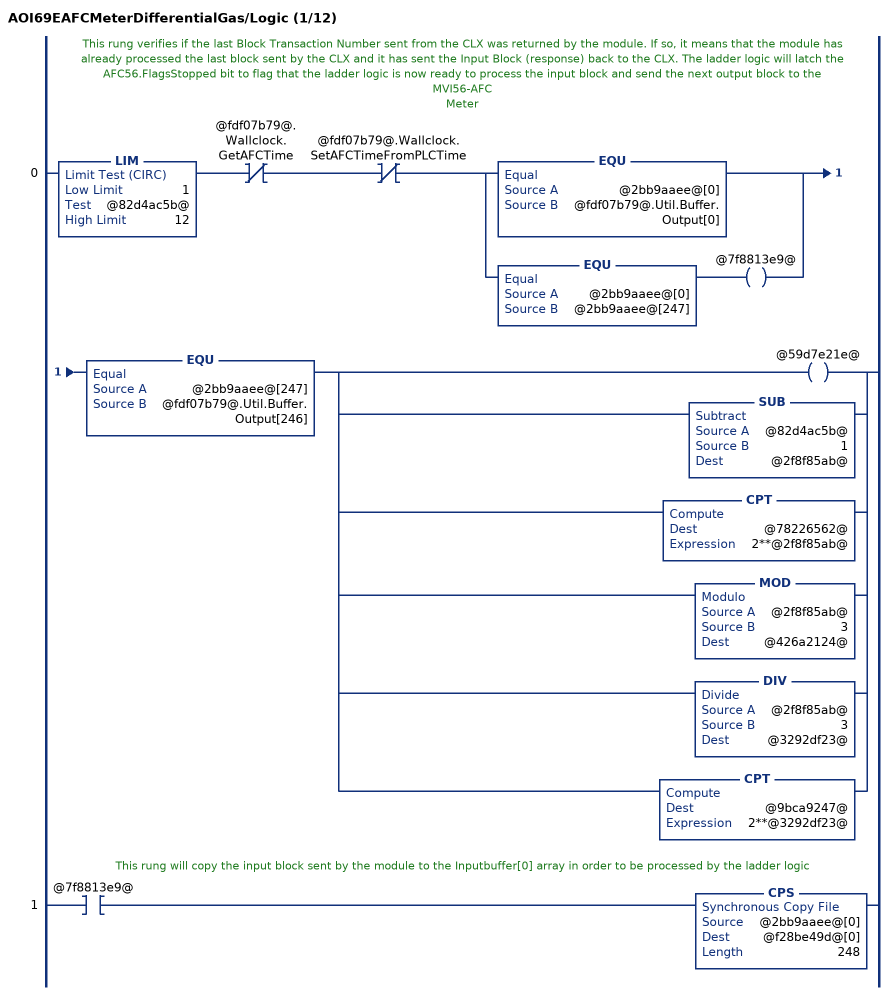
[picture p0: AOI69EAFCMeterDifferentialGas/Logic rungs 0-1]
   // This rung verifies if the last Block Transaction Number sent from the CLX was returned by the module. If so, it means that the module has already processed the last block sent by the CLX and it has sent the Input Block (response) back to the CLX. The ladder logic will latch the AFC56.FlagsStopped bit to flag that the ladder logic is now ready to process the input block and send the next output block to the MVI56-AFC
   // Meter
   0: LIM(1,@82d4ac5b@,12)XIO(@fdf07b79@.Wallclock.GetAFCTime)XIO(@fdf07b79@.Wallclock.SetAFCTimeFromPLCTime)[EQU(@2bb9aaee@[0],@fdf07b79@.Util.Buffer.Output[0]) ,EQU(@2bb9aaee@[0],@2bb9aaee@[247]) OTE(@7f8813e9@) ]EQU(@2bb9aaee@[247],@fdf07b79@.Util.Buffer.Output[246])[OTE(@59d7e21e@) ,SUB(@82d4ac5b@,1,@2f8f85ab@) ,CPT(@78226562@,2**@2f8f85ab@) ,MOD(@2f8f85ab@,3,@426a2124@) ,DIV(@2f8f85ab@,3,@3292df23@) ,CPT(@9bca9247@,2**@3292df23@) ];
   // This rung will copy the input block sent by the module to the Inputbuffer[0] array in order to be processed by the ladder logic
   1: XIC(@7f8813e9@)CPS(@2bb9aaee@[0],@f28be49d@[0],248);
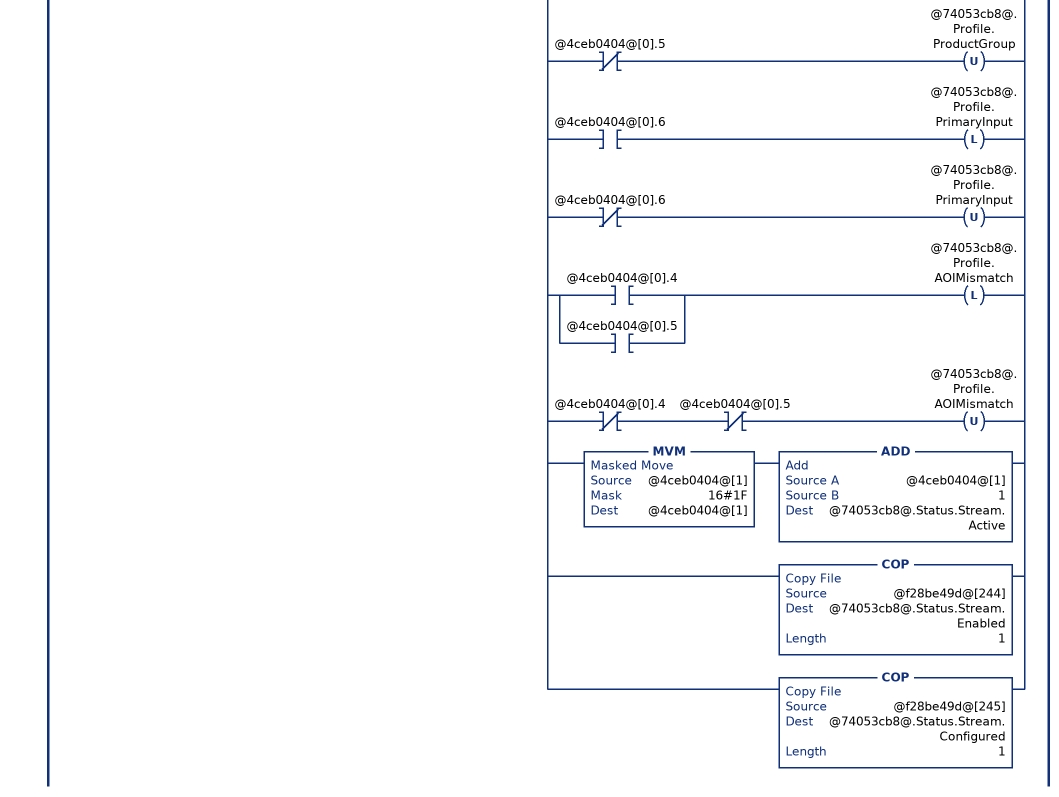
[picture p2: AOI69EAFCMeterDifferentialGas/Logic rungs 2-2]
   // Read process input backplane return and
   // meter profile (when block ID matches meter number).
   2: XIC(@7f8813e9@)LIM(1,@f28be49d@[0],12)[COP(@f28be49d@[3+@2f8f85ab@*15],@74053cb8@.BackPlaneReturn.StandardRaw[0],14) ,COP(@74053cb8@.BackPlaneReturn.StandardRaw[0],@74053cb8@.BackPlaneReturn.StandardDefault,1) ,COP(@f28be49d@[246],@fdf07b79@.SiteStatus,1) ,EQU(@f28be49d@[0],@82d4ac5b@) [COP(@f28be49d@[243],@4ceb0404@[0],2) ,[XIC(@4ceb0404@[0].0) OTL(@74053cb8@.Status.Meter.EnableAlarm) ,XIO(@4ceb0404@[0].0) OTU(@74053cb8@.Status.Meter.EnableAlarm) ] ,[XIC(@4ceb0404@[0].1) OTL(@74053cb8@.Status.Meter.Enabled) ,XIO(@4ceb0404@[0].1) OTU(@74053cb8@.Status.Meter.Enabled) ] ,[[XIC(@4ceb0404@[0].4) OTL(@74053cb8@.Profile.MeterType) ,XIO(@4ceb0404@[0].4) OTU(@74053cb8@.Profile.MeterType) ] ,[XIC(@4ceb0404@[0].5) OTL(@74053cb8@.Profile.ProductGroup) ,XIO(@4ceb0404@[0].5) OTU(@74053cb8@.Profile.ProductGroup) ] ,[XIC(@4ceb0404@[0].6) OTL(@74053cb8@.Profile.PrimaryInput) ,XIO(@4ceb0404@[0].6) OTU(@74053cb8@.Profile.PrimaryInput) ] ] ,[[XIC(@4ceb0404@[0].4) ,XIC(@4ceb0404@[0].5) ] OTL(@74053cb8@.Profile.AOIMismatch) ,XIO(@4ceb0404@[0].4) XIO(@4ceb0404@[0].5) OTU(@74053cb8@.Profile.AOIMismatch) ] ,MVM(@4ceb0404@[1],16#1F,@4ceb0404@[1]) ADD(@4ceb0404@[1],1,@74053cb8@.Status.Stream.Active) ,COP(@f28be49d@[244],@74053cb8@.Status.Stream.Enabled,1) ,COP(@f28be49d@[245],@74053cb8@.Status.Stream.Configured,1) ] ];
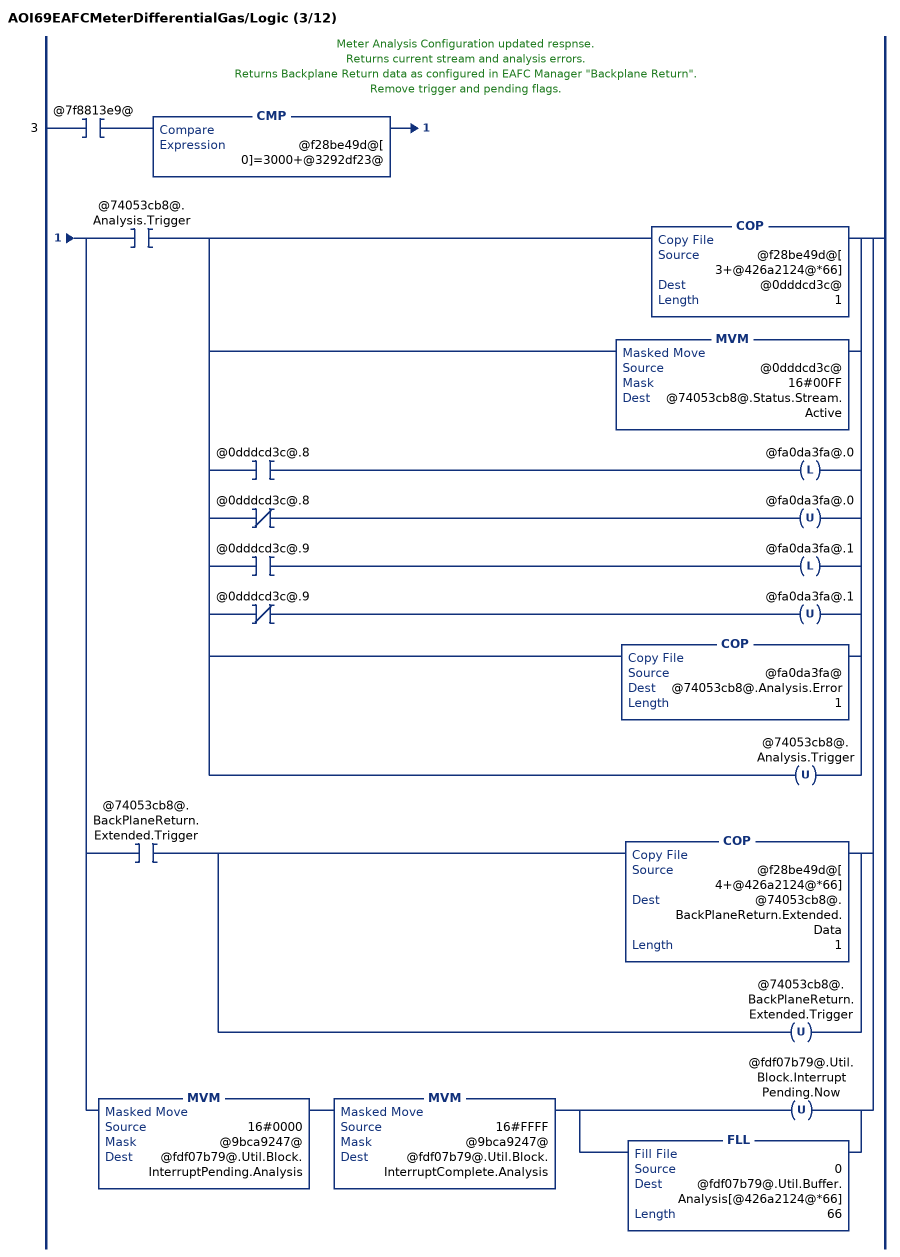
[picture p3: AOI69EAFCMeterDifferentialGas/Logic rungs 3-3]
   // Meter Analysis Configuration updated respnse.
   // Returns current stream and analysis errors.
   // Returns Backplane Return data as configured in EAFC Manager "Backplane Return".
   // Remove trigger and pending flags.
   3: XIC(@7f8813e9@)CMP(@f28be49d@[0]=3000+@3292df23@)[XIC(@74053cb8@.Analysis.Trigger) [COP(@f28be49d@[3+@426a2124@*66],@0dddcd3c@,1) ,MVM(@0dddcd3c@,16#00FF,@74053cb8@.Status.Stream.Active) ,[XIC(@0dddcd3c@.8) OTL(@fa0da3fa@.0) ,XIO(@0dddcd3c@.8) OTU(@fa0da3fa@.0) ] ,[XIC(@0dddcd3c@.9) OTL(@fa0da3fa@.1) ,XIO(@0dddcd3c@.9) OTU(@fa0da3fa@.1) ] ,COP(@fa0da3fa@,@74053cb8@.Analysis.Error,1) ,OTU(@74053cb8@.Analysis.Trigger) ] ,XIC(@74053cb8@.BackPlaneReturn.Extended.Trigger) [COP(@f28be49d@[4+@426a2124@*66],@74053cb8@.BackPlaneReturn.Extended.Data,1) ,OTU(@74053cb8@.BackPlaneReturn.Extended.Trigger) ] ,MVM(16#0000,@9bca9247@,@fdf07b79@.Util.Block.InterruptPending.Analysis) MVM(16#FFFF,@9bca9247@,@fdf07b79@.Util.Block.InterruptComplete.Analysis) [OTU(@fdf07b79@.Util.Block.InterruptPending.Now) ,FLL(0,@fdf07b79@.Util.Buffer.Analysis[@426a2124@*66],66) ] ];
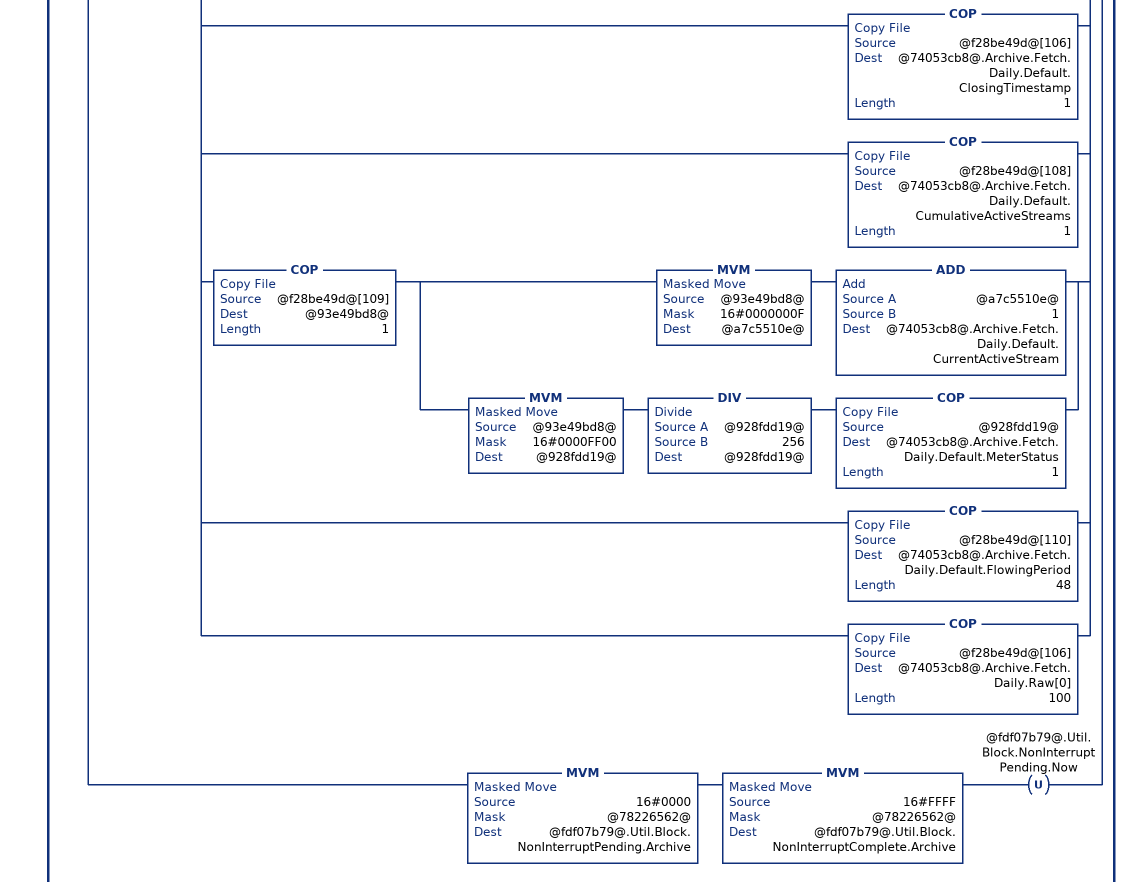
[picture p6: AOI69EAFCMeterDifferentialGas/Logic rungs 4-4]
   // Archive Fetch to default and raw UDT's.
   // Get archive alarms.
   // Remove trigger and pending flags.
   4: XIC(@7f8813e9@)CMP(@f28be49d@[0]=6000+@2f8f85ab@)[XIC(@74053cb8@.Archive.Fetch.Hourly.Trigger) [OTU(@74053cb8@.Archive.Fetch.Hourly.Trigger) ,[[XIC(@f28be49d@[3].0) OTL(@74053cb8@.Archive.Fetch.Hourly.Error.ArchiveSelectionInvalid) ,XIO(@f28be49d@[3].0) OTU(@74053cb8@.Archive.Fetch.Hourly.Error.ArchiveSelectionInvalid) ] ,[XIC(@f28be49d@[3].1) OTL(@74053cb8@.Archive.Fetch.Hourly.Error.AgeOutsideSize) ,XIO(@f28be49d@[3].1) OTU(@74053cb8@.Archive.Fetch.Hourly.Error.AgeOutsideSize) ] ,[XIC(@f28be49d@[3].2) OTL(@74053cb8@.Archive.Fetch.Hourly.Error.ArchiveNeverWritten) ,XIO(@f28be49d@[3].2) OTU(@74053cb8@.Archive.Fetch.Hourly.Error.ArchiveNeverWritten) ] ] ,COP(@f28be49d@[4],@74053cb8@.Archive.Fetch.Hourly.Default.ClosingTimestamp,1) ,COP(@f28be49d@[6],@74053cb8@.Archive.Fetch.Hourly.Default.CumulativeActiveStreams,1) ,COP(@f28be49d@[7],@93e49bd8@,1) [MVM(@93e49bd8@,16#0000000F,@a7c5510e@) ADD(@a7c5510e@,1,@74053cb8@.Archive.Fetch.Hourly.Default.CurrentActiveStream) ,MVM(@93e49bd8@,16#0000FF00,@928fdd19@) DIV(@928fdd19@,256,@928fdd19@) COP(@928fdd19@,@74053cb8@.Archive.Fetch.Hourly.Default.MeterStatus,1) ] ,COP(@f28be49d@[8],@74053cb8@.Archive.Fetch.Hourly.Default.FlowingPeriod,48) ,COP(@f28be49d@[4],@74053cb8@.Archive.Fetch.Hourly.Raw[0],100) ] ,XIC(@74053cb8@.Archive.Fetch.Daily.Trigger) [OTU(@74053cb8@.Archive.Fetch.Daily.Trigger) ,[[XIC(@f28be49d@[105].0) OTL(@74053cb8@.Archive.Fetch.Daily.Error.ArchiveSelectionInvalid) ,XIO(@f28be49d@[105].0) OTU(@74053cb8@.Archive.Fetch.Daily.Error.ArchiveSelectionInvalid) ] ,[XIC(@f28be49d@[105].1) OTL(@74053cb8@.Archive.Fetch.Daily.Error.AgeOutsideSize) ,XIO(@f28be49d@[105].1) OTU(@74053cb8@.Archive.Fetch.Daily.Error.AgeOutsideSize) ] ,[XIC(@f28be49d@[105].2) OTL(@74053cb8@.Archive.Fetch.Daily.Error.ArchiveNeverWritten) ,XIO(@f28be49d@[105].2) OTU(@74053cb8@.Archive.Fetch.Daily.Error.ArchiveNeverWritten) ] ] ,COP(@f28be49d@[106],@74053cb8@.Archive.Fetch.Daily.Default.ClosingTimestamp,1) ,COP(@f28be49d@[108],@74053cb8@.Archive.Fetch.Daily.Default.CumulativeActiveStreams,1) ,COP(@f28be49d@[109],@93e49bd8@,1) [MVM(@93e49bd8@,16#0000000F,@a7c5510e@) ADD(@a7c5510e@,1,@74053cb8@.Archive.Fetch.Daily.Default.CurrentActiveStream) ,MVM(@93e49bd8@,16#0000FF00,@928fdd19@) DIV(@928fdd19@,256,@928fdd19@) COP(@928fdd19@,@74053cb8@.Archive.Fetch.Daily.Default.MeterStatus,1) ] ,COP(@f28be49d@[110],@74053cb8@.Archive.Fetch.Daily.Default.FlowingPeriod,48) ,COP(@f28be49d@[106],@74053cb8@.Archive.Fetch.Daily.Raw[0],100) ] ,MVM(16#0000,@78226562@,@fdf07b79@.Util.Block.NonInterruptPending.Archive) MVM(16#FFFF,@78226562@,@fdf07b79@.Util.Block.NonInterruptComplete.Archive) OTU(@fdf07b79@.Util.Block.NonInterruptPending.Now) ];
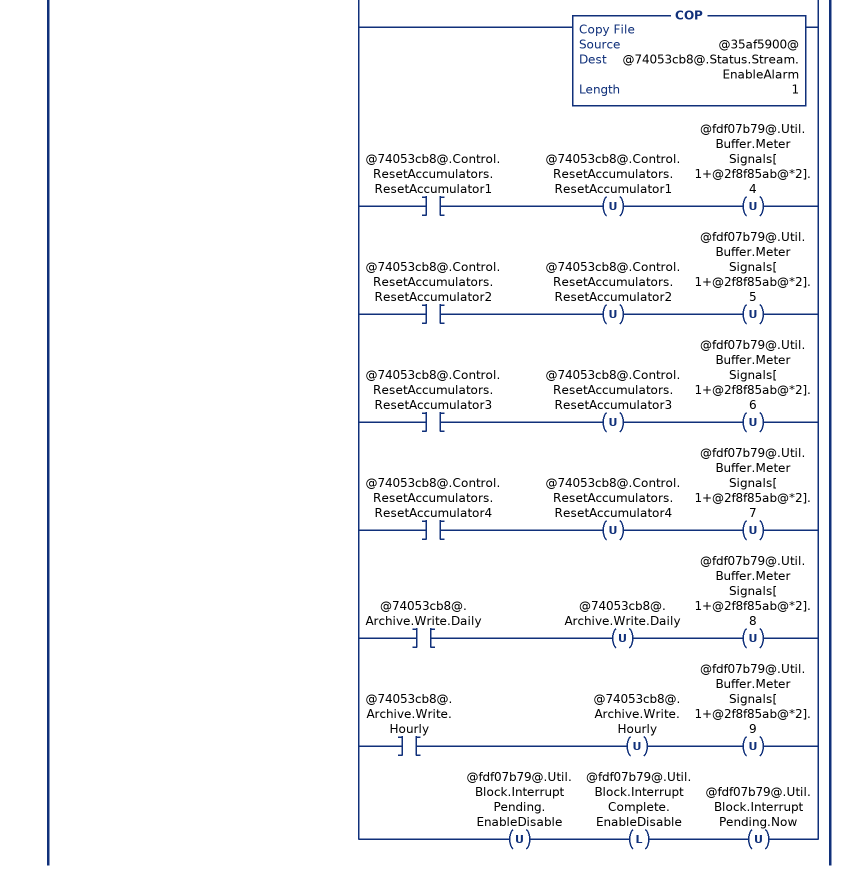
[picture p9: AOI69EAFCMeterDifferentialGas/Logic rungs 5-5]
   // Meter status and stream status.
   // Remove trigger and pending flags.
   5: XIC(@7f8813e9@)EQU(@f28be49d@[0],7000)[[MVM(@f28be49d@[3],@78226562@,@09ff9d4f@) ,[NEQ(@09ff9d4f@,0) OTL(@74053cb8@.Status.Meter.Enabled) ,EQU(@09ff9d4f@,0) OTU(@74053cb8@.Status.Meter.Enabled) ] ,OTU(@74053cb8@.Control.Meter.Enable) MVM(16#0000,@78226562@,@fdf07b79@.Util.Buffer.MeterEnableDisable[1]) ,OTU(@74053cb8@.Control.Meter.Disable) MVM(16#0000,@78226562@,@fdf07b79@.Util.Buffer.MeterEnableDisable[3]) ] ,[XIC(@74053cb8@.Control.Stream.EnableSelected) [COP(@f28be49d@[7+@2f8f85ab@*3],@74053cb8@.Status.Stream.Enabled,1) ,COP(@f28be49d@[8+@2f8f85ab@*3],@74053cb8@.Status.Stream.Configured,1) ,OTU(@74053cb8@.Control.Stream.EnableSelected) OTU(@74053cb8@.Control.Stream.DisableSelected) ] ,XIC(@74053cb8@.Control.Stream.DisableSelected) [COP(@f28be49d@[55+@2f8f85ab@*3],@74053cb8@.Status.Stream.Enabled,1) ,COP(@f28be49d@[56+@2f8f85ab@*3],@74053cb8@.Status.Stream.Configured,1) ,OTU(@74053cb8@.Control.Stream.EnableSelected) OTU(@74053cb8@.Control.Stream.DisableSelected) ] ] ,[OTU(@74053cb8@.Control.Stream.SetSelectedToActive) ,COP(@f28be49d@[103+@2f8f85ab@*2],@0dddcd3c@,1) ,[XIC(@0dddcd3c@.8) OTL(@35af5900@.0) ,XIO(@0dddcd3c@.8) OTU(@35af5900@.0) ] ,[XIC(@0dddcd3c@.9) OTL(@35af5900@.1) ,XIO(@0dddcd3c@.9) OTU(@35af5900@.1) ] ,[XIC(@0dddcd3c@.10) OTL(@35af5900@.2) ,XIO(@0dddcd3c@.10) OTU(@35af5900@.2) ] ,[XIC(@0dddcd3c@.11) OTL(@35af5900@.3) ,XIO(@0dddcd3c@.11) OTU(@35af5900@.3) ] ,MVM(@0dddcd3c@,16#000F,@3f536ccd@) ADD(@3f536ccd@,1,@74053cb8@.Status.Stream.Active) ,COP(@35af5900@,@74053cb8@.Status.Stream.EnableAlarm,1) ] ,[XIC(@74053cb8@.Control.ResetAccumulators.ResetAccumulator1) OTU(@74053cb8@.Control.ResetAccumulators.ResetAccumulator1) OTU(@fdf07b79@.Util.Buffer.MeterSignals[1+@2f8f85ab@*2].4) ,XIC(@74053cb8@.Control.ResetAccumulators.ResetAccumulator2) OTU(@74053cb8@.Control.ResetAccumulators.ResetAccumulator2) OTU(@fdf07b79@.Util.Buffer.MeterSignals[1+@2f8f85ab@*2].5) ,XIC(@74053cb8@.Control.ResetAccumulators.ResetAccumulator3) OTU(@74053cb8@.Control.ResetAccumulators.ResetAccumulator3) OTU(@fdf07b79@.Util.Buffer.MeterSignals[1+@2f8f85ab@*2].6) ,XIC(@74053cb8@.Control.ResetAccumulators.ResetAccumulator4) OTU(@74053cb8@.Control.ResetAccumulators.ResetAccumulator4) OTU(@fdf07b79@.Util.Buffer.MeterSignals[1+@2f8f85ab@*2].7) ,XIC(@74053cb8@.Archive.Write.Daily) OTU(@74053cb8@.Archive.Write.Daily) OTU(@fdf07b79@.Util.Buffer.MeterSignals[1+@2f8f85ab@*2].8) ,XIC(@74053cb8@.Archive.Write.Hourly) OTU(@74053cb8@.Archive.Write.Hourly) OTU(@fdf07b79@.Util.Buffer.MeterSignals[1+@2f8f85ab@*2].9) ] ,OTU(@fdf07b79@.Util.Block.InterruptPending.EnableDisable) OTL(@fdf07b79@.Util.Block.InterruptComplete.EnableDisable) OTU(@fdf07b79@.Util.Block.InterruptPending.Now) ];
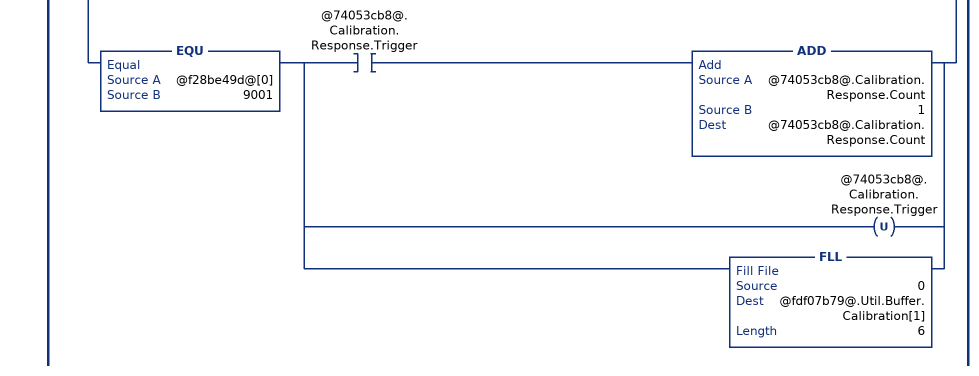
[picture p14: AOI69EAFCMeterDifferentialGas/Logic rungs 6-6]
   // Meter transmitter calibration.
   6: XIC(@7f8813e9@)[EQU(@f28be49d@[0],9000) ,EQU(@f28be49d@[0],9001) ][MVM(@f28be49d@[3],16#0F00,@c7ddefd3@) ,DIV(@c7ddefd3@,16#100,@c7ddefd3@) ]EQU(@c7ddefd3@,@2f8f85ab@)XIO(@f28be49d@[3].14)[EQU(@f28be49d@[0],9000) [XIO(@a9249fea@) ADD(@74053cb8@.Calibration.Request.Count,1,@74053cb8@.Calibration.Request.Count) ,OTL(@a9249fea@) [COP(@f28be49d@[3],@5b497894@,1) ,MVM(@5b497894@,16#000F,@179c6a05@) ] ,[EQU(@179c6a05@,0) [OTL(@74053cb8@.Calibration.Request.ProcessVariable.DifferentialPressure) ,OTU(@74053cb8@.Calibration.Request.ProcessVariable.Temperature) ,OTU(@74053cb8@.Calibration.Request.ProcessVariable.Pressure) ] ,EQU(@179c6a05@,1) [OTL(@74053cb8@.Calibration.Request.ProcessVariable.Temperature) ,OTU(@74053cb8@.Calibration.Request.ProcessVariable.DifferentialPressure) ,OTU(@74053cb8@.Calibration.Request.ProcessVariable.Pressure) ] ,EQU(@179c6a05@,2) [OTL(@74053cb8@.Calibration.Request.ProcessVariable.Pressure) ,OTU(@74053cb8@.Calibration.Request.ProcessVariable.DifferentialPressure) ,OTU(@74053cb8@.Calibration.Request.ProcessVariable.Temperature) ] ] ,[[XIC(@f28be49d@[5].2) [OTL(@74053cb8@.Calibration.Request.ActionType.ZeroShift) ,COP(@f28be49d@[6],@74053cb8@.Calibration.Request.Value.ZeroShift.Applied,2) ] ,XIO(@f28be49d@[5].2) [OTU(@74053cb8@.Calibration.Request.ActionType.ZeroShift) ,FLL(0,@74053cb8@.Calibration.Request.Value.ZeroShift.Applied,2) ] ] ,[XIC(@f28be49d@[5].3) [OTL(@74053cb8@.Calibration.Request.ActionType.SetZero) ,COP(@f28be49d@[10],@74053cb8@.Calibration.Request.Value.SetZero.Applied,2) ] ,XIO(@f28be49d@[5].3) [OTU(@74053cb8@.Calibration.Request.ActionType.SetZero) ,FLL(0,@74053cb8@.Calibration.Request.Value.SetZero.Applied,2) ] ] ,[XIC(@f28be49d@[5].4) [OTL(@74053cb8@.Calibration.Request.ActionType.SetSpan) ,COP(@f28be49d@[14],@74053cb8@.Calibration.Request.Value.SetSpan.Applied,2) ] ,XIO(@f28be49d@[5].4) [OTU(@74053cb8@.Calibration.Request.ActionType.SetSpan) ,FLL(0,@74053cb8@.Calibration.Request.Value.SetSpan.Applied,2) ] ] ,[XIC(@f28be49d@[5].5) [OTL(@74053cb8@.Calibration.Request.ActionType.SetMid1) ,COP(@f28be49d@[18],@74053cb8@.Calibration.Request.Value.SetMid1.Applied,2) ] ,XIO(@f28be49d@[5].5) [OTU(@74053cb8@.Calibration.Request.ActionType.SetMid1) ,FLL(0,@74053cb8@.Calibration.Request.Value.SetMid1.Applied,2) ] ] ,[XIC(@f28be49d@[5].6) [OTL(@74053cb8@.Calibration.Request.ActionType.SetMid2) ,COP(@f28be49d@[22],@74053cb8@.Calibration.Request.Value.SetMid2.Applied,2) ] ,XIO(@f28be49d@[5].6) [OTU(@74053cb8@.Calibration.Request.ActionType.SetMid2) ,FLL(0,@74053cb8@.Calibration.Request.Value.SetMid2.Applied,2) ] ] ,[XIC(@f28be49d@[5].7) [OTL(@74053cb8@.Calibration.Request.ActionType.SetMid3) ,COP(@f28be49d@[26],@74053cb8@.Calibration.Request.Value.SetMid3.Applied,2) ] ,XIO(@f28be49d@[5].7) [OTU(@74053cb8@.Calibration.Request.ActionType.SetMid3) ,FLL(0,@74053cb8@.Calibration.Request.Value.SetMid3.Applied,2) ] ] ] ] ,EQU(@f28be49d@[0],9001) [XIC(@74053cb8@.Calibration.Response.Trigger) ADD(@74053cb8@.Calibration.Response.Count,1,@74053cb8@.Calibration.Response.Count) ,OTU(@74053cb8@.Calibration.Response.Trigger) ,FLL(0,@fdf07b79@.Util.Buffer.Calibration[1],6) ] ];
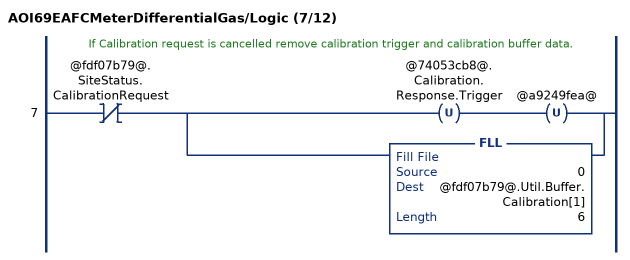
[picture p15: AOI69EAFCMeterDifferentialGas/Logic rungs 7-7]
   // If Calibration request is cancelled remove calibration trigger and calibration buffer data.
   7: XIO(@fdf07b79@.SiteStatus.CalibrationRequest)[OTU(@74053cb8@.Calibration.Response.Trigger) OTU(@a9249fea@) ,FLL(0,@fdf07b79@.Util.Buffer.Calibration[1],6) ];
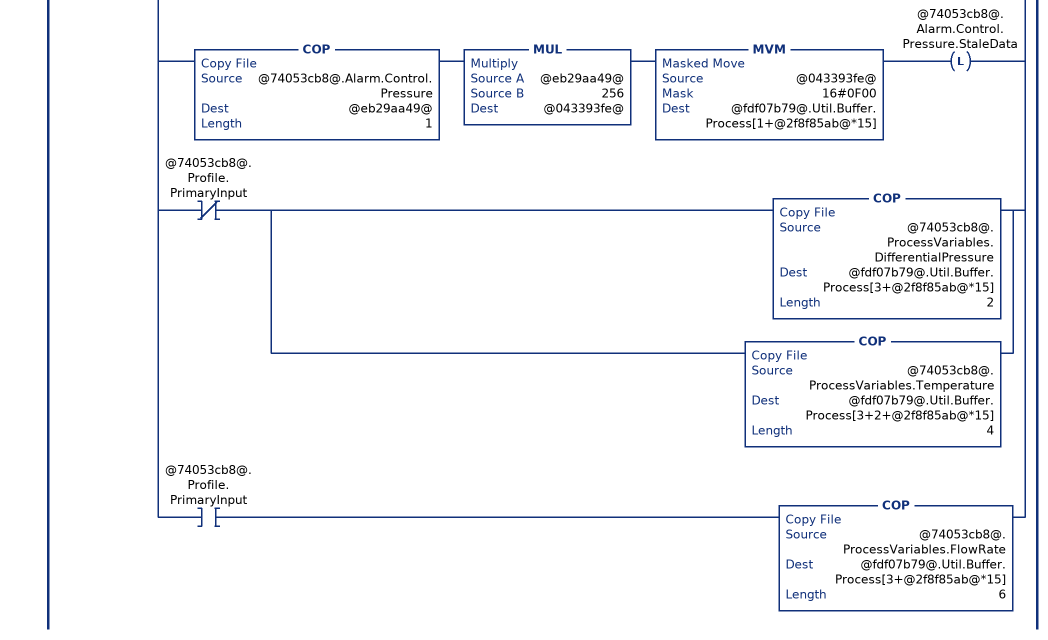
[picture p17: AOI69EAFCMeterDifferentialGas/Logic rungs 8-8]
   // Process variables and process alarms to send to module.
   8: XIC(@59d7e21e@)[ADD(16#A000,@82d4ac5b@,@9881d5f7@) COP(@9881d5f7@,@fdf07b79@.Util.Buffer.Process[@2f8f85ab@*15],1) ,[XIO(@74053cb8@.Profile.PrimaryInput) XIC(@74053cb8@.Alarm.Control.DifferentialPressure.SetAutoClearStaleData) OTU(@74053cb8@.Alarm.Control.DifferentialPressure.StaleData) ,XIC(@74053cb8@.Profile.PrimaryInput) XIC(@74053cb8@.Alarm.Control.FlowRate.SetAutoClearStaleData) OTU(@74053cb8@.Alarm.Control.FlowRate.StaleData) ,XIO(@74053cb8@.Profile.PrimaryInput) COP(@74053cb8@.Alarm.Control.DifferentialPressure,@fdf07b79@.Util.Buffer.Process[1+@2f8f85ab@*15],1) OTL(@74053cb8@.Alarm.Control.DifferentialPressure.StaleData) ,XIC(@74053cb8@.Profile.PrimaryInput) COP(@74053cb8@.Alarm.Control.FlowRate,@fdf07b79@.Util.Buffer.Process[1+@2f8f85ab@*15],1) OTL(@74053cb8@.Alarm.Control.FlowRate.StaleData) ] ,[XIC(@74053cb8@.Alarm.Control.Temperature.SetAutoClearStaleData) OTU(@74053cb8@.Alarm.Control.Temperature.StaleData) ,COP(@74053cb8@.Alarm.Control.Temperature,@eb29aa49@,1) MUL(@eb29aa49@,16,@043393fe@) MVM(@043393fe@,16#00F0,@fdf07b79@.Util.Buffer.Process[1+@2f8f85ab@*15]) OTL(@74053cb8@.Alarm.Control.Temperature.StaleData) ] ,[XIC(@74053cb8@.Alarm.Control.Pressure.SetAutoClearStaleData) OTU(@74053cb8@.Alarm.Control.Pressure.StaleData) ,COP(@74053cb8@.Alarm.Control.Pressure,@eb29aa49@,1) MUL(@eb29aa49@,256,@043393fe@) MVM(@043393fe@,16#0F00,@fdf07b79@.Util.Buffer.Process[1+@2f8f85ab@*15]) OTL(@74053cb8@.Alarm.Control.Pressure.StaleData) ] ,XIO(@74053cb8@.Profile.PrimaryInput) [COP(@74053cb8@.ProcessVariables.DifferentialPressure,@fdf07b79@.Util.Buffer.Process[3+@2f8f85ab@*15],2) ,COP(@74053cb8@.ProcessVariables.Temperature,@fdf07b79@.Util.Buffer.Process[3+2+@2f8f85ab@*15],4) ] ,XIC(@74053cb8@.Profile.PrimaryInput) COP(@74053cb8@.ProcessVariables.FlowRate,@fdf07b79@.Util.Buffer.Process[3+@2f8f85ab@*15],6) ];
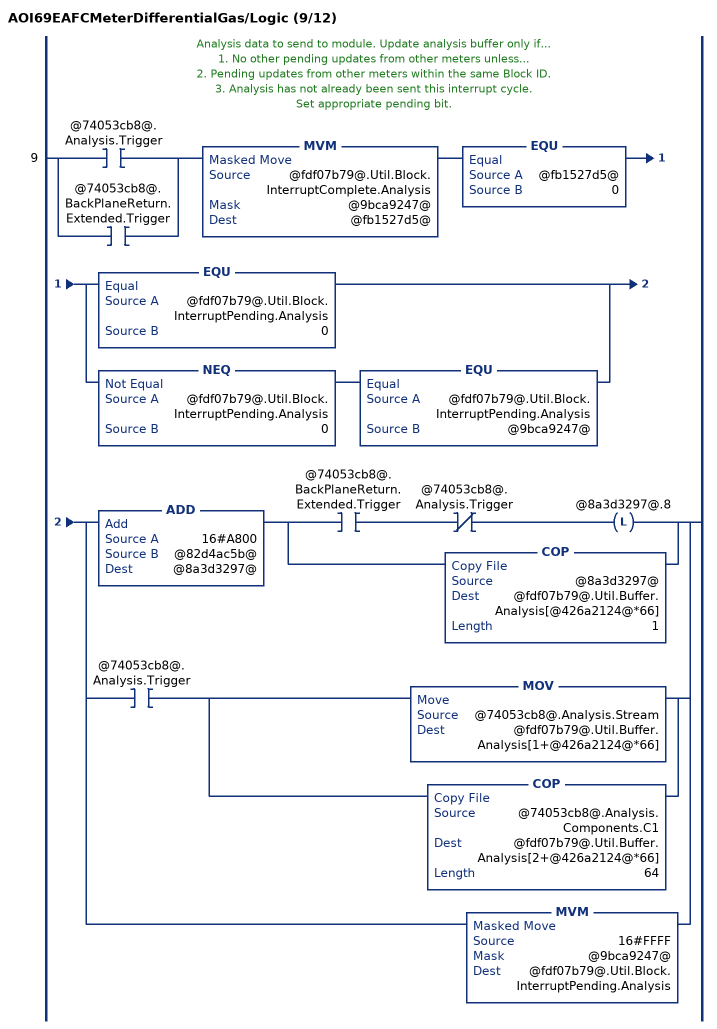
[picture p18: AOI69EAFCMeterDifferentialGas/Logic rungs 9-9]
   // Analysis data to send to module. Update analysis buffer only if...
   // 1. No other pending updates from other meters unless...
   // 2. Pending updates from other meters within the same Block ID.
   // 3. Analysis has not already been sent this interrupt cycle.
   // Set appropriate pending bit.
   9: [XIC(@74053cb8@.Analysis.Trigger) ,XIC(@74053cb8@.BackPlaneReturn.Extended.Trigger) ]MVM(@fdf07b79@.Util.Block.InterruptComplete.Analysis,@9bca9247@,@fb1527d5@)EQU(@fb1527d5@,0)[EQU(@fdf07b79@.Util.Block.InterruptPending.Analysis,0) ,NEQ(@fdf07b79@.Util.Block.InterruptPending.Analysis,0) EQU(@fdf07b79@.Util.Block.InterruptPending.Analysis,@9bca9247@) ][ADD(16#A800,@82d4ac5b@,@8a3d3297@) [XIC(@74053cb8@.BackPlaneReturn.Extended.Trigger) XIO(@74053cb8@.Analysis.Trigger) OTL(@8a3d3297@.8) ,COP(@8a3d3297@,@fdf07b79@.Util.Buffer.Analysis[@426a2124@*66],1) ] ,XIC(@74053cb8@.Analysis.Trigger) [MOV(@74053cb8@.Analysis.Stream,@fdf07b79@.Util.Buffer.Analysis[1+@426a2124@*66]) ,COP(@74053cb8@.Analysis.Components.C1,@fdf07b79@.Util.Buffer.Analysis[2+@426a2124@*66],64) ] ,MVM(16#FFFF,@9bca9247@,@fdf07b79@.Util.Block.InterruptPending.Analysis) ];
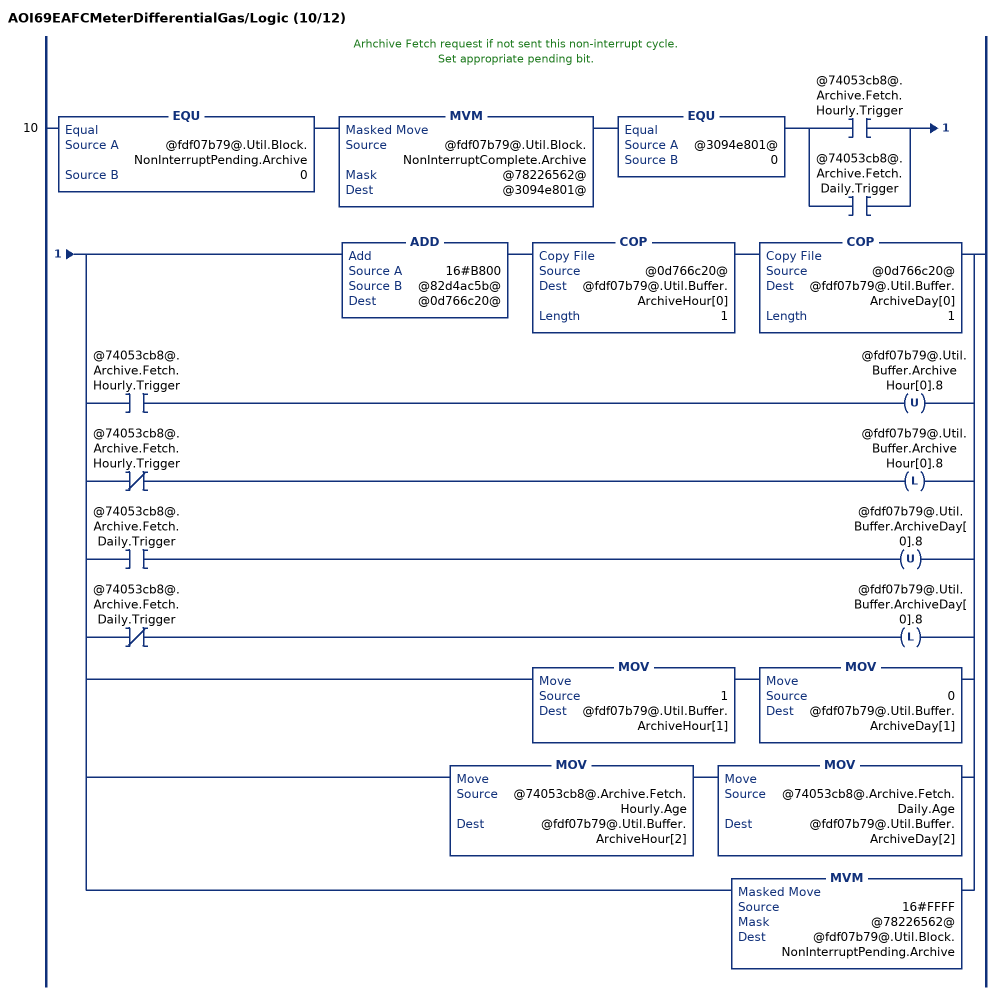
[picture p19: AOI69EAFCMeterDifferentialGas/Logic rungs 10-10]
   // Arhchive Fetch request if not sent this non-interrupt cycle.
   // Set appropriate pending bit.
   10: EQU(@fdf07b79@.Util.Block.NonInterruptPending.Archive,0)MVM(@fdf07b79@.Util.Block.NonInterruptComplete.Archive,@78226562@,@3094e801@)EQU(@3094e801@,0)[XIC(@74053cb8@.Archive.Fetch.Hourly.Trigger) ,XIC(@74053cb8@.Archive.Fetch.Daily.Trigger) ][ADD(16#B800,@82d4ac5b@,@0d766c20@) COP(@0d766c20@,@fdf07b79@.Util.Buffer.ArchiveHour[0],1) COP(@0d766c20@,@fdf07b79@.Util.Buffer.ArchiveDay[0],1) ,[XIC(@74053cb8@.Archive.Fetch.Hourly.Trigger) OTU(@fdf07b79@.Util.Buffer.ArchiveHour[0].8) ,XIO(@74053cb8@.Archive.Fetch.Hourly.Trigger) OTL(@fdf07b79@.Util.Buffer.ArchiveHour[0].8) ] ,[XIC(@74053cb8@.Archive.Fetch.Daily.Trigger) OTU(@fdf07b79@.Util.Buffer.ArchiveDay[0].8) ,XIO(@74053cb8@.Archive.Fetch.Daily.Trigger) OTL(@fdf07b79@.Util.Buffer.ArchiveDay[0].8) ] ,MOV(1,@fdf07b79@.Util.Buffer.ArchiveHour[1]) MOV(0,@fdf07b79@.Util.Buffer.ArchiveDay[1]) ,MOV(@74053cb8@.Archive.Fetch.Hourly.Age,@fdf07b79@.Util.Buffer.ArchiveHour[2]) MOV(@74053cb8@.Archive.Fetch.Daily.Age,@fdf07b79@.Util.Buffer.ArchiveDay[2]) ,MVM(16#FFFF,@78226562@,@fdf07b79@.Util.Block.NonInterruptPending.Archive) ];
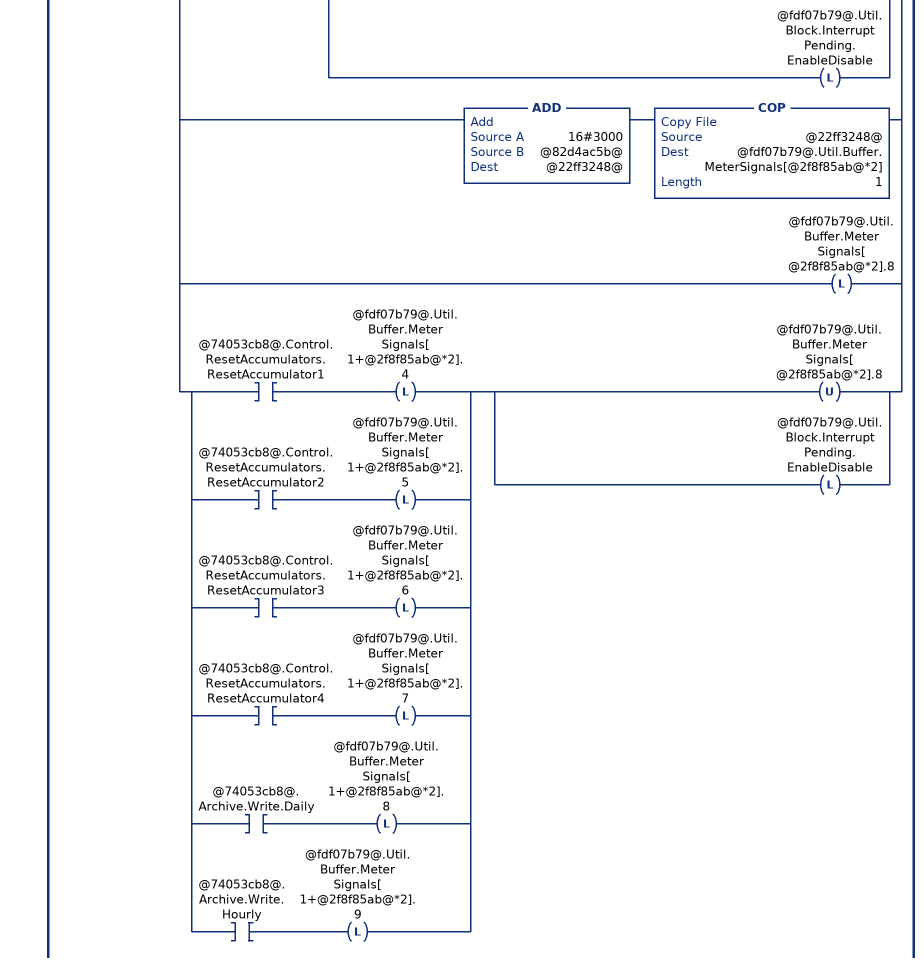
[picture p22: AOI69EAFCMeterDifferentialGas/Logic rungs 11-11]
   // Meter Enable.
   // Meter Disable.
   // Stream Select.
   // Stream Enable.
   // Stream Disable.
   // Set pending bit if not set this interrupt cycle.
   11: XIO(@fdf07b79@.Util.Block.InterruptComplete.EnableDisable)[LIM(1,@74053cb8@.Control.Stream.Selected,16) CPT(@86f42fda@,2**(@74053cb8@.Control.Stream.Selected-1)) ,[XIC(@74053cb8@.Control.Meter.Enable) MVM(16#FFFF,@78226562@,@fdf07b79@.Util.Buffer.MeterEnableDisable[1]) MVM(16#0000,@78226562@,@fdf07b79@.Util.Buffer.MeterEnableDisable[3]) ,XIC(@74053cb8@.Control.Meter.Disable) MVM(16#FFFF,@78226562@,@fdf07b79@.Util.Buffer.MeterEnableDisable[3]) MVM(16#0000,@78226562@,@fdf07b79@.Util.Buffer.MeterEnableDisable[1]) ] OTL(@fdf07b79@.Util.Block.InterruptPending.EnableDisable) ,[ADD(16#CC00,@82d4ac5b@,@037da483@) COP(@037da483@,@fdf07b79@.Util.Buffer.StreamEnable[@2f8f85ab@*3],1) ,XIO(@74053cb8@.Control.Stream.EnableSelected) OTL(@fdf07b79@.Util.Buffer.StreamEnable[@2f8f85ab@*3].8) ,XIC(@74053cb8@.Control.Stream.EnableSelected) [OTU(@fdf07b79@.Util.Buffer.StreamEnable[@2f8f85ab@*3].8) ,COP(@86f42fda@,@fdf07b79@.Util.Buffer.StreamEnable[1+@2f8f85ab@*3],1) ,OTL(@fdf07b79@.Util.Block.InterruptPending.EnableDisable) ] ] ,[ADD(16#C800,@82d4ac5b@,@96e67035@) COP(@96e67035@,@fdf07b79@.Util.Buffer.StreamDisable[@2f8f85ab@*3],1) ,XIO(@74053cb8@.Control.Stream.DisableSelected) OTL(@fdf07b79@.Util.Buffer.StreamDisable[@2f8f85ab@*3].8) ,XIC(@74053cb8@.Control.Stream.DisableSelected) [OTU(@fdf07b79@.Util.Buffer.StreamDisable[@2f8f85ab@*3].8) ,COP(@86f42fda@,@fdf07b79@.Util.Buffer.StreamDisable[1+@2f8f85ab@*3],1) ,OTL(@fdf07b79@.Util.Block.InterruptPending.EnableDisable) ] ] ,[ADD(16#3C00,@82d4ac5b@,@8f49b4f6@) COP(@8f49b4f6@,@fdf07b79@.Util.Buffer.StreamSelect[@2f8f85ab@*2],1) ,XIO(@74053cb8@.Control.Stream.SetSelectedToActive) OTL(@fdf07b79@.Util.Buffer.StreamSelect[@2f8f85ab@*2].8) ,XIC(@74053cb8@.Control.Stream.SetSelectedToActive) [OTU(@fdf07b79@.Util.Buffer.StreamSelect[@2f8f85ab@*2].8) ,MOV(@74053cb8@.Control.Stream.Selected,@fdf07b79@.Util.Buffer.StreamSelect[1+@2f8f85ab@*2]) ,OTL(@fdf07b79@.Util.Block.InterruptPending.EnableDisable) ] ] ,[ADD(16#3000,@82d4ac5b@,@22ff3248@) COP(@22ff3248@,@fdf07b79@.Util.Buffer.MeterSignals[@2f8f85ab@*2],1) ,OTL(@fdf07b79@.Util.Buffer.MeterSignals[@2f8f85ab@*2].8) ,[XIC(@74053cb8@.Control.ResetAccumulators.ResetAccumulator1) OTL(@fdf07b79@.Util.Buffer.MeterSignals[1+@2f8f85ab@*2].4) ,XIC(@74053cb8@.Control.ResetAccumulators.ResetAccumulator2) OTL(@fdf07b79@.Util.Buffer.MeterSignals[1+@2f8f85ab@*2].5) ,XIC(@74053cb8@.Control.ResetAccumulators.ResetAccumulator3) OTL(@fdf07b79@.Util.Buffer.MeterSignals[1+@2f8f85ab@*2].6) ,XIC(@74053cb8@.Control.ResetAccumulators.ResetAccumulator4) OTL(@fdf07b79@.Util.Buffer.MeterSignals[1+@2f8f85ab@*2].7) ,XIC(@74053cb8@.Archive.Write.Daily) OTL(@fdf07b79@.Util.Buffer.MeterSignals[1+@2f8f85ab@*2].8) ,XIC(@74053cb8@.Archive.Write.Hourly) OTL(@fdf07b79@.Util.Buffer.MeterSignals[1+@2f8f85ab@*2].9) ] [OTU(@fdf07b79@.Util.Buffer.MeterSignals[@2f8f85ab@*2].8) ,OTL(@fdf07b79@.Util.Block.InterruptPending.EnableDisable) ] ] ];
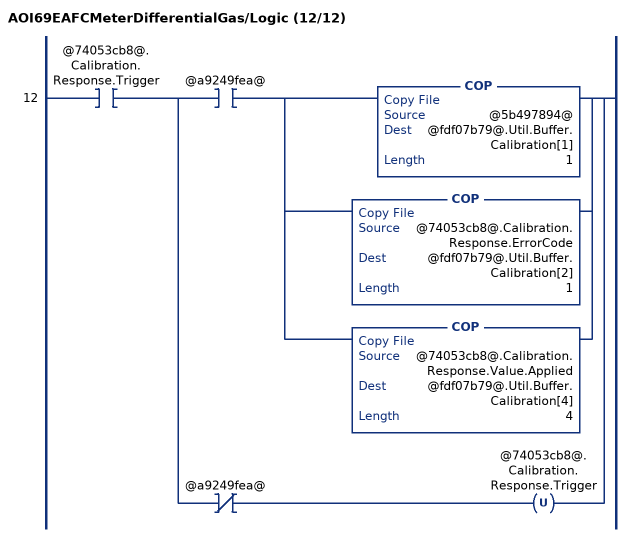
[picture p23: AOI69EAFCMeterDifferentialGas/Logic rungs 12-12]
   12: XIC(@74053cb8@.Calibration.Response.Trigger)[XIC(@a9249fea@) [COP(@5b497894@,@fdf07b79@.Util.Buffer.Calibration[1],1) ,COP(@74053cb8@.Calibration.Response.ErrorCode,@fdf07b79@.Util.Buffer.Calibration[2],1) ,COP(@74053cb8@.Calibration.Response.Value.Applied,@fdf07b79@.Util.Buffer.Calibration[4],4) ] ,XIO(@a9249fea@) OTU(@74053cb8@.Calibration.Response.Trigger) ];
END_ROUTINE

ROUTINE Prescan   (* ladder *)
// Prescan
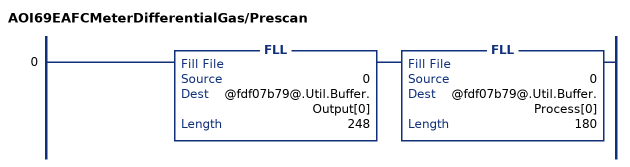
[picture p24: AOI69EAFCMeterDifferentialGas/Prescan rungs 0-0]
   0: FLL(0,@fdf07b79@.Util.Buffer.Output[0],248)FLL(0,@fdf07b79@.Util.Buffer.Process[0],180);
END_ROUTINE
END_ADD_ON_INSTRUCTION

VAR_GLOBAL   (* controller tags *)
   Local:1:I : AB:1756_MODULE_INT_496Bytes:I:0;
   AFC : AFCEModuleDef;
   AFCMeter01DifferentialGas : AFCEMeterDifferentialGas;
   AOI69EAFCMeter01DifferentialGas : AOI69EAFCMeterDifferentialGas;
END_VAR

PROGRAM MainProgram

ROUTINE MainRoutine   (* ladder *)
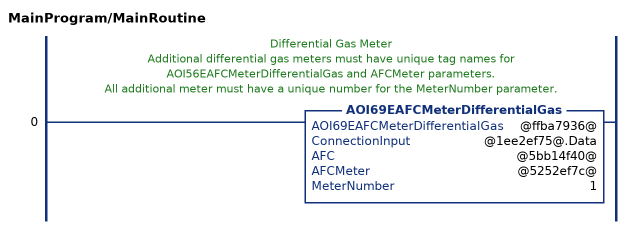
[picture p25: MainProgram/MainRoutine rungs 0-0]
   // Differential Gas Meter
   // Additional differential gas meters must have unique tag names for AOI56EAFCMeterDifferentialGas and AFCMeter parameters.
   // All additional meter must have a unique number for the MeterNumber parameter.
   0: AOI69EAFCMeterDifferentialGas(@ffba7936@,@1ee2ef75@.Data,@5bb14f40@,@5252ef7c@,1);
END_ROUTINE
END_PROGRAM
